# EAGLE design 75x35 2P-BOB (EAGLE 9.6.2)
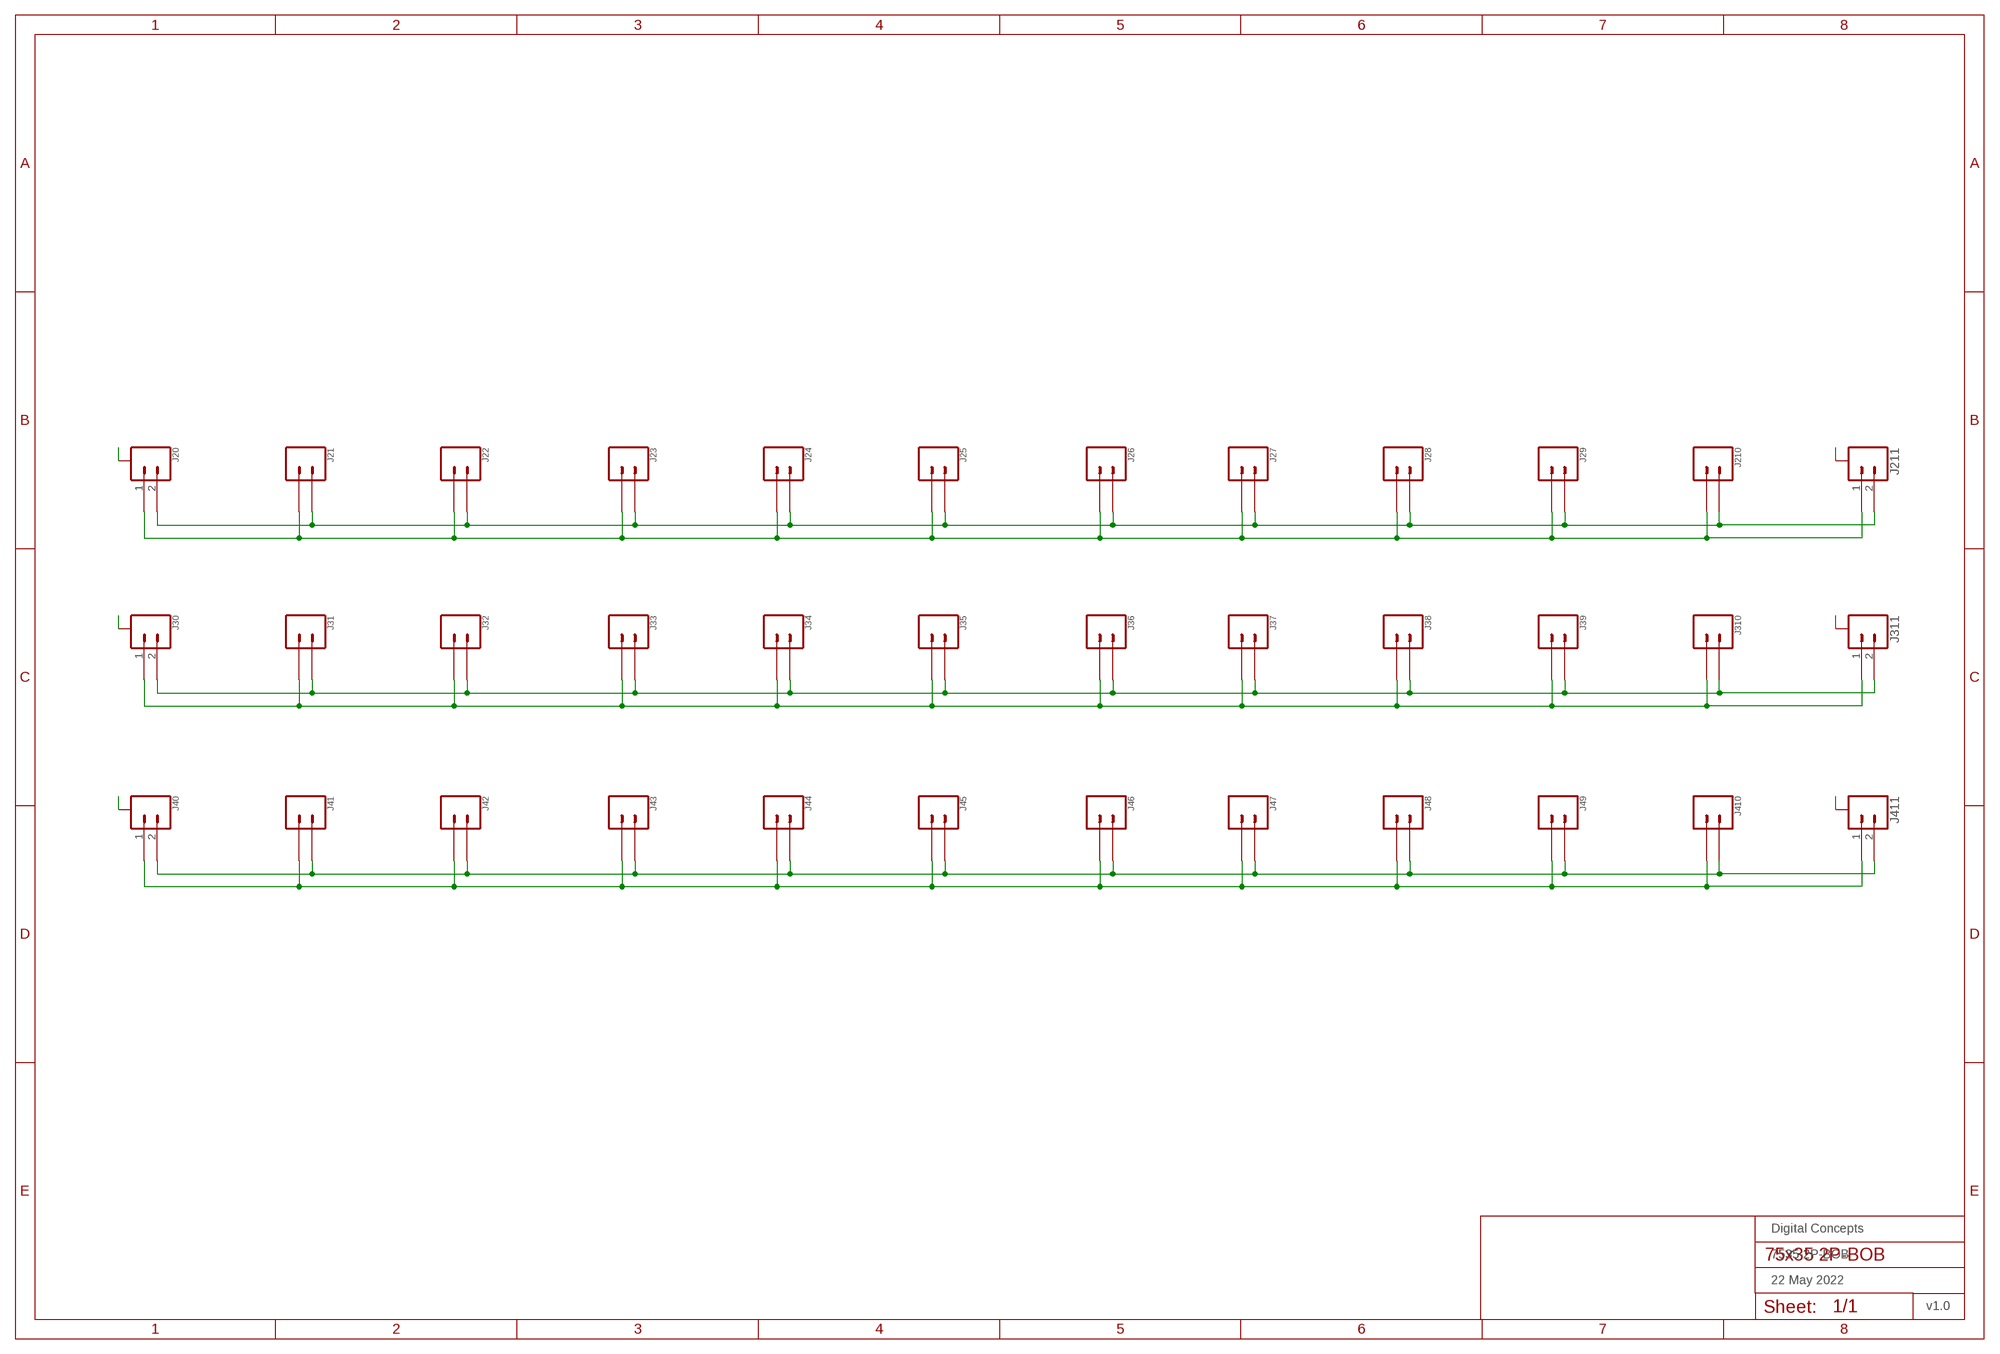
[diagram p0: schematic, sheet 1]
FRAME1 (FRAME-A3L-LOC): DATE: 22 May 2022; OWNER: Digital Concepts; TITLE: 7535-2P-BOB; VERSION: v1.0

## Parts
J20  JST-SH1.0-2-SMD-VERTICAL  [JST-SH1.0-2-VERTICAL]
J21  JST-GH1.25-2-VERTICAL  [JST-GH1.25-2-VERTICAL]
J22  JST-PH2.0-2-VERTICAL  [JST-PH2.0-2-VERTICAL]
J23  HEADER-1X2-GENERIC  [CONN_02-GENERIC]
J24  HEADER-1X2-GENERIC  [CONN_02-GENERIC]
J25  HEADER-1X2-GENERIC  [CONN_02-GENERIC]
J26  HEADER-1X2-GENERIC  [CONN_02-GENERIC]
J27  HEADER-1X2-GENERIC  [CONN_02-GENERIC]
J28  HEADER-1X2-GENERIC  [CONN_02-GENERIC]
J29  JST-PH2.0-2-VERTICAL  [JST-PH2.0-2-VERTICAL]
J30  JST-SH1.0-2-SMD-VERTICAL  [JST-SH1.0-2-VERTICAL]
J31  JST-GH1.25-2-VERTICAL  [JST-GH1.25-2-VERTICAL]
J32  JST-PH2.0-2-VERTICAL  [JST-PH2.0-2-VERTICAL]
J33  HEADER-1X2-GENERIC  [CONN_02-GENERIC]
J34  HEADER-1X2-GENERIC  [CONN_02-GENERIC]
J35  HEADER-1X2-GENERIC  [CONN_02-GENERIC]
J36  HEADER-1X2-GENERIC  [CONN_02-GENERIC]
J37  HEADER-1X2-GENERIC  [CONN_02-GENERIC]
J38  HEADER-1X2-GENERIC  [CONN_02-GENERIC]
J39  JST-PH2.0-2-VERTICAL  [JST-PH2.0-2-VERTICAL]
J40  JST-SH1.0-2-SMD-VERTICAL  [JST-SH1.0-2-VERTICAL]
J41  JST-GH1.25-2-VERTICAL  [JST-GH1.25-2-VERTICAL]
J42  JST-PH2.0-2-VERTICAL  [JST-PH2.0-2-VERTICAL]
J43  HEADER-1X2-GENERIC  [CONN_02-GENERIC]
J44  HEADER-1X2-GENERIC  [CONN_02-GENERIC]
J45  HEADER-1X2-GENERIC  [CONN_02-GENERIC]
J46  HEADER-1X2-GENERIC  [CONN_02-GENERIC]
J47  HEADER-1X2-GENERIC  [CONN_02-GENERIC]
J48  HEADER-1X2-GENERIC  [CONN_02-GENERIC]
J49  JST-PH2.0-2-VERTICAL  [JST-PH2.0-2-VERTICAL]
J210  JST-GH1.25-2-VERTICAL  [JST-GH1.25-2-VERTICAL]
J211  JST-SH1.0-2-SMD-VERTICAL  [JST-SH1.0-2-VERTICAL]
J310  JST-GH1.25-2-VERTICAL  [JST-GH1.25-2-VERTICAL]
J311  JST-SH1.0-2-SMD-VERTICAL  [JST-SH1.0-2-VERTICAL]
J410  JST-GH1.25-2-VERTICAL  [JST-GH1.25-2-VERTICAL]
J411  JST-SH1.0-2-SMD-VERTICAL  [JST-SH1.0-2-VERTICAL]

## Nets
A: J20.A@1(A) J20.A@2(A) J30.A@1(A) J30.A@2(A) J40.A@1(A) J40.A@2(A) J211.A@1(A) J211.A@2(A) J311.A@1(A) J311.A@2(A) J411.A@1(A) J411.A@2(A)
N$1: J20.1 J21.1 J22.1 J23.1 J24.1 J25.1 J26.1 J27.1 J28.1 J29.1 J210.1 J211.1
N$2: J30.2 J31.2 J32.2 J33.2 J34.2 J35.2 J36.2 J37.2 J38.2 J39.2 J310.2 J311.2
N$3: J30.1 J31.1 J32.1 J33.1 J34.1 J35.1 J36.1 J37.1 J38.1 J39.1 J310.1 J311.1
N$4: J40.2 J41.2 J42.2 J43.2 J44.2 J45.2 J46.2 J47.2 J48.2 J49.2 J410.2 J411.2
N$5: J40.1 J41.1 J42.1 J43.1 J44.1 J45.1 J46.1 J47.1 J48.1 J49.1 J410.1 J411.1
N$7: J20.2 J21.2 J22.2 J23.2 J24.2 J25.2 J26.2 J27.2 J28.2 J29.2 J210.2 J211.2

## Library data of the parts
J20 J30 J40 J211 J311 J411 = digitalconcepts:JST-SH1.0-2-SMD-VERTICAL: JST SH1.0 2P SMD Vertical Connector
J21 J31 J41 J210 J310 J410 = digitalconcepts:JST-GH1.25-2-VERTICAL: JST GH1.25 2P PTH Connector
J22 J29 J32 J39 J42 J49 = digitalconcepts:JST-PH2.0-2-VERTICAL: PH2.0 2P Vertical Connector
J23-J28 J33-J38 J43-J48 = digitalconcepts:HEADER-1X2-GENERIC: Single Row 2-Pin Header

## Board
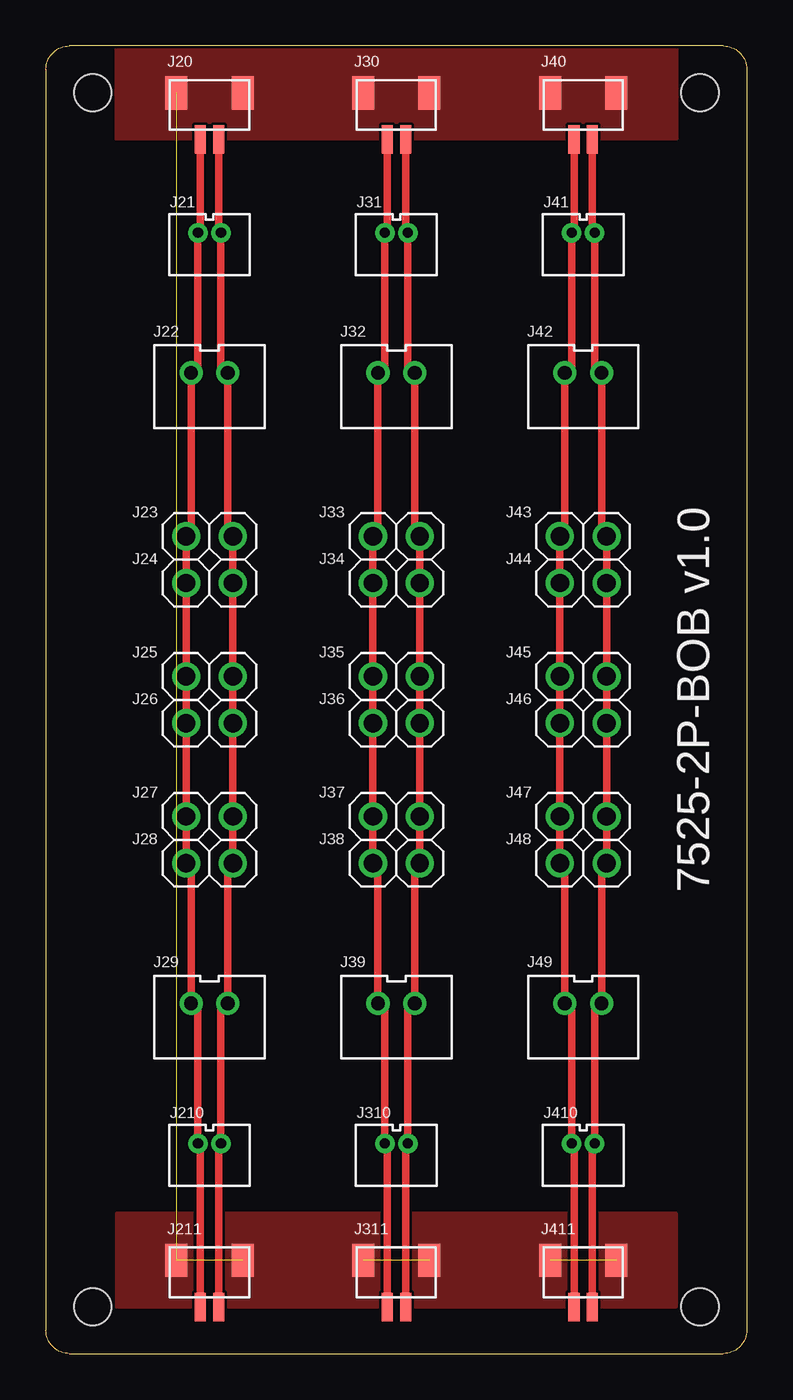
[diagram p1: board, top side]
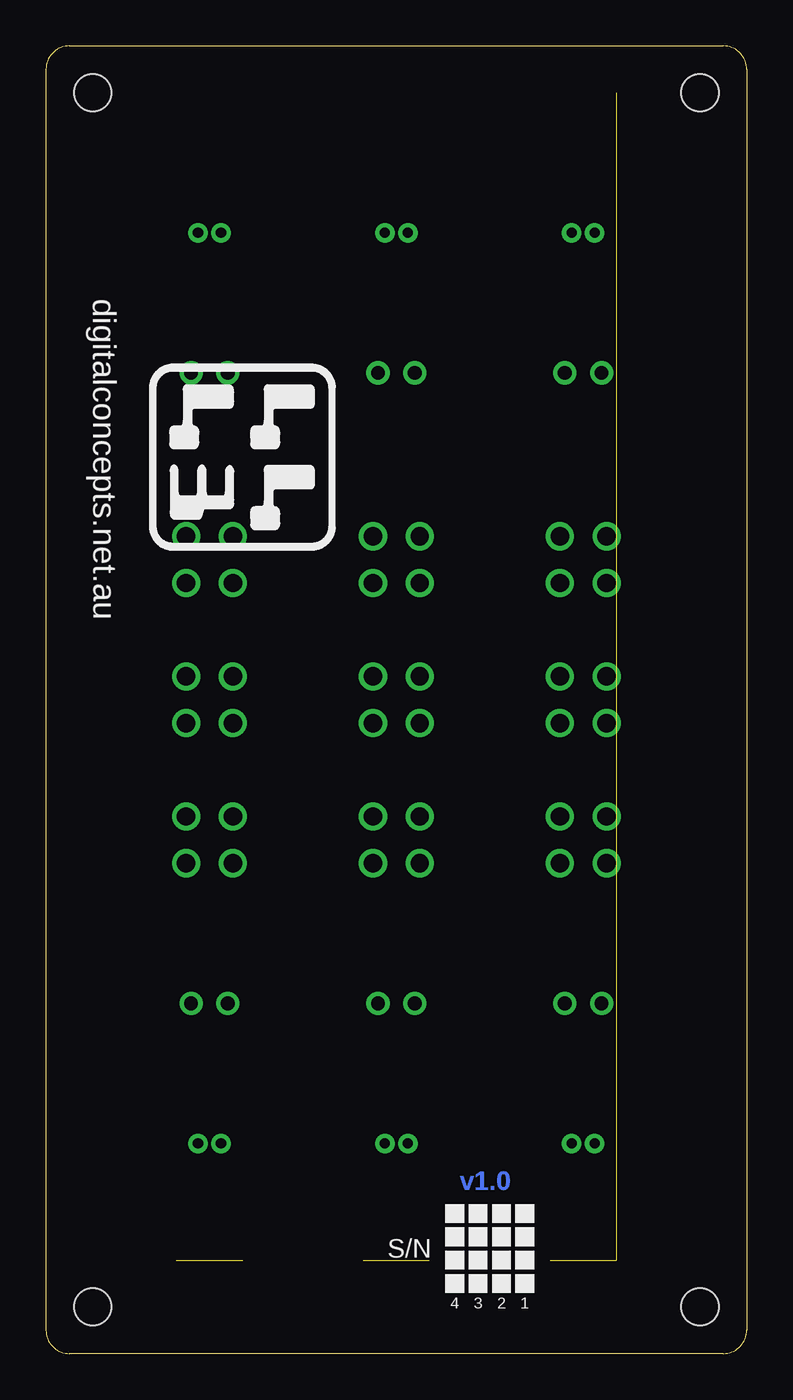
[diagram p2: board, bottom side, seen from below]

Size 38.1 x 71.12 mm. Coordinates in mm from the lower left corner, seen from the top.
Outline: 36.83,71.12 arc-90 38.1,69.85 38.1,1.27 arc-90 36.83,0 1.27,0 arc-90 0,1.27 0,69.85 arc-90 1.27,71.12 36.83,71.12
Copper layers (1*16): Top 0.035mm / dielectric 1.5mm / Bottom 0.035mm
Design rules "default *": minimum track width 6mil, minimum drill 0.35mm, track to track 6mil, track to pad 6mil, pad to pad 6mil, via to via 6mil, smd to smd 6mil, copper to edge 6mil, drill to drill 6mil, minimum pad ring 10mil, minimum via ring 8mil, stop-mask expansion 4mil, vias tented up to drill 0mil, thermal gap 0mil
Holes 2.03 mm at 2.54,68.58 2.54,2.54 35.56,2.54 35.56,68.58

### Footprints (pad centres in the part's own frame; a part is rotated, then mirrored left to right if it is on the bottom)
JST-SH1.0-2-VERTICAL = smd 0.6 x 1.55: 1 -0.5,-2.54; 2 0.5,-2.54 | smd 1.2 x 1.8: A@1 -1.8,-0.015; A@2 1.8,-0.015
JST-GH1.25-2-VERTICAL = drill 0.55 pad 1.016: 1 -0.625,0; 2 0.625,0
JST-PH2.0-2-VERTICAL = drill 0.75: 1 -1,0; 2 1,0
CONN_02-GENERIC = drill 1 pad 1.524: 1 0,0; 2 2.54,0

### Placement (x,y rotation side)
J20  8.89,68.58 0 top
J21  8.89,60.96 0 top
J22  8.89,53.34 0 top
J23  7.62,44.45 0 top
J24  7.62,41.91 0 top
J25  7.62,36.83 0 top
J26  7.62,34.29 0 top
J27  7.62,29.21 0 top
J28  7.62,26.67 0 top
J29  8.89,19.05 0 top
J30  19.05,68.58 0 top
J31  19.05,60.96 0 top
J32  19.05,53.34 0 top
J33  17.78,44.45 0 top
J34  17.78,41.91 0 top
J35  17.78,36.83 0 top
J36  17.78,34.29 0 top
J37  17.78,29.21 0 top
J38  17.78,26.67 0 top
J39  19.05,19.05 0 top
J40  29.21,68.58 0 top
J41  29.21,60.96 0 top
J42  29.21,53.34 0 top
J43  27.94,44.45 0 top
J44  27.94,41.91 0 top
J45  27.94,36.83 0 top
J46  27.94,34.29 0 top
J47  27.94,29.21 0 top
J48  27.94,26.67 0 top
J49  29.21,19.05 0 top
J210  8.89,11.43 0 top
J211  8.89,5.08 0 top
J310  19.05,11.43 0 top
J311  19.05,5.08 0 top
J410  29.21,11.43 0 top
J411  29.21,5.08 0 top

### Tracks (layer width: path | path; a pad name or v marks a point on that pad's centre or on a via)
A  (4 unrouted)
  pour Top: 3.81,71.12 34.29,71.12 34.29,66.04 3.81,66.04
  pour Top: 3.81,2.54 34.29,2.54 34.29,7.62 3.81,7.62
N$1
  Top 0.406: J20.1 8.39,61.09 J21.1 8.27,53.72 J22.1 7.89,44.72 J23.1 J24.1 J25.1 J26.1 J27.1 J28.1 7.89,26.4 J29.1 8.27,18.68 J210.1 8.39,11.3 J211.1
N$2
  Top 0.406: J30.2 19.55,61.09 J31.2 19.68,53.72 J32.2 20.05,44.72 J33.2 J34.2 J35.2 J36.2 J37.2 J38.2 20.05,26.4 J39.2 19.68,18.68 J310.2 19.55,11.3 J311.2
N$3
  Top 0.406: J30.1 18.55,61.09 J31.1 18.43,53.72 J32.1 18.05,44.72 J33.1 J34.1 J35.1 J36.1 J37.1 J38.1 18.05,26.4 J39.1 18.43,18.68 J310.1 18.55,11.3 J311.1
N$4
  Top 0.406: J40.2 29.71,61.09 J41.2 29.84,53.72 J42.2 30.21,44.72 J43.2 J44.2 J45.2 J46.2 J47.2 J48.2 30.21,26.4 J49.2 29.84,18.68 J410.2 29.71,11.3 J411.2
N$5
  Top 0.406: J40.1 28.71,61.09 J41.1 28.59,53.72 J42.1 28.21,44.72 J43.1 J44.1 J45.1 J46.1 J47.1 J48.1 28.21,26.4 J49.1 28.59,18.68 J410.1 28.71,11.3 J411.1
N$7
  Top 0.406: J20.2 9.39,61.09 J21.2 9.52,53.72 J22.2 9.89,44.72 J23.2 J24.2 J25.2 J26.2 J27.2 J28.2 9.89,26.4 J29.2 9.52,18.68 J210.2 9.39,11.3 J211.2

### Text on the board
Bottom: v1.0
tPlace: 7525-2P-BOB v1.0
bPlace: digitalconcepts.net.au | S/N | 1 | 2 | 3 | 4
